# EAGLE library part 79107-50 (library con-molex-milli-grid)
RECEPTACAL
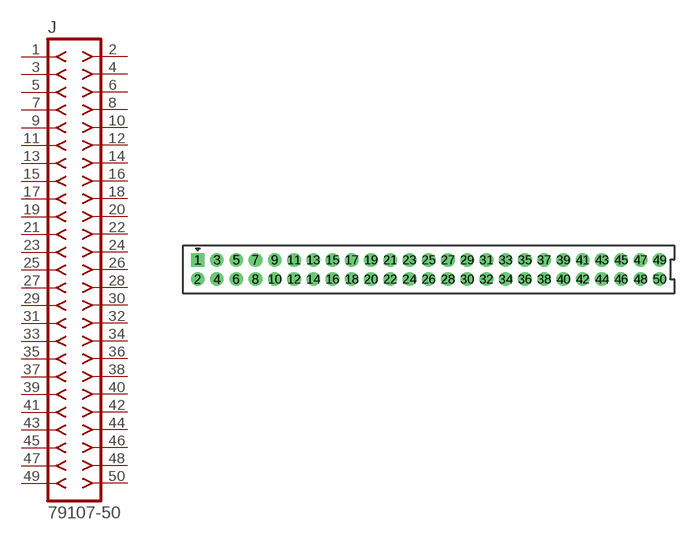
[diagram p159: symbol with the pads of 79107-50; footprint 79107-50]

Designator prefix J

## 79107-50  [79107-50]
1  1  pas
2  2  pas
3  3  pas
4  4  pas
5  5  pas
6  6  pas
7  7  pas
8  8  pas
9  9  pas
10  10  pas
11  11  pas
12  12  pas
13  13  pas
14  14  pas
15  15  pas
16  16  pas
17  17  pas
18  18  pas
19  19  pas
20  20  pas
21  21  pas
22  22  pas
23  23  pas
24  24  pas
25  25  pas
26  26  pas
27  27  pas
28  28  pas
29  29  pas
30  30  pas
31  31  pas
32  32  pas
33  33  pas
34  34  pas
35  35  pas
36  36  pas
37  37  pas
38  38  pas
39  39  pas
40  40  pas
41  41  pas
42  42  pas
43  43  pas
44  44  pas
45  45  pas
46  46  pas
47  47  pas
48  48  pas
49  49  pas
50  50  pas

## Footprint 79107-50 (pad centres in mm)
RECEPTACAL Dual Row, Vertical, Through-Hole
drill 0.914 square: 1 -24,1
drill 0.914: 2 -24,-1; 3 -22,1; 4 -22,-1; 5 -20,1; 6 -20,-1; 7 -18,1; 8 -18,-1; 9 -16,1; 10 -16,-1; 11 -14,1; 12 -14,-1; 13 -12,1; 14 -12,-1; 15 -10,1; 16 -10,-1; 17 -8,1; 18 -8,-1; 19 -6,1; 20 -6,-1; 21 -4,1; 22 -4,-1; 23 -2,1; 24 -2,-1; 25 0,1; 26 0,-1; 27 2,1; 28 2,-1; 29 4,1; 30 4,-1; 31 6,1; 32 6,-1; 33 8,1; 34 8,-1; 35 10,1; 36 10,-1; 37 12,1; 38 12,-1; 39 14,1; 40 14,-1; 41 16,1; 42 16,-1; 43 18,1; 44 18,-1; 45 20,1; 46 20,-1; 47 22,1; 48 22,-1; 49 24,1; 50 24,-1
